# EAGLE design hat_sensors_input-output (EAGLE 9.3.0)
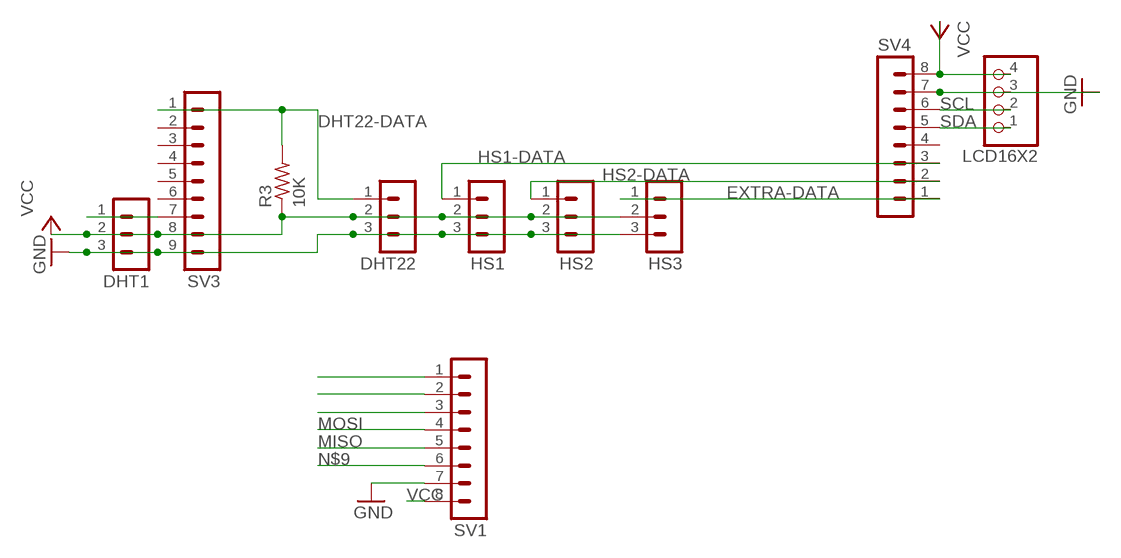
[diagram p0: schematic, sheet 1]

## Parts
DHT1  MA03-1  [MA03-1]
DHT22  MA03-1  [MA03-1]
HS1  MA03-1  [MA03-1]
HS2  MA03-1  [MA03-1]
HS3  MA03-1  [MA03-1]
LCD16X2  PINHD-1X4  [1X04]
R3  10K  RES-US1206  [R1206]
SV1  MA08-1  [MA08-1]
SV3  MA09-1  [MA09-1]
SV4  MA08-1  [MA08-1]

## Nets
DHT22-DATA: DHT22.1 R3.2 SV3.1
EXTRA-DATA: HS3.1 SV4.1
GND: DHT1.3 DHT22.3 HS1.3 HS2.3 HS3.3 LCD16X2.3 SV1.7 SV3.9 SV4.7
HS1-DATA: HS1.1 SV4.3
HS2-DATA: HS2.1 SV4.2
MISO: SV1.5
MOSI: SV1.4
N$2: SV1.1
N$4: DHT1.1 SV3.7
N$9: SV1.6
N$17: SV1.2
N$18: SV1.3
SCL: LCD16X2.2 SV4.6
SDA: LCD16X2.1 SV4.5
VCC: DHT1.2 DHT22.2 HS1.2 HS2.2 HS3.2 LCD16X2.4 R3.1 SV1.8 SV3.8 SV4.8
Unconnected: SV3.2 SV3.3 SV3.4 SV3.5 SV3.6 SV4.4

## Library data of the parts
DHT1 DHT22 HS1-HS3 = con-lstb:MA03-1: PIN HEADER; OC_FARNELL: unknown; OC_NEWARK: unknown
LCD16X2 = pinhead:PINHD-1X4: PIN HEADER
R3 = fab:RES-US: Resistor (US Symbol)
SV1 SV4 = con-lstb:MA08-1: PIN HEADER
SV3 = con-lstb:MA09-1: PIN HEADER; OC_FARNELL: unknown; OC_NEWARK: unknown

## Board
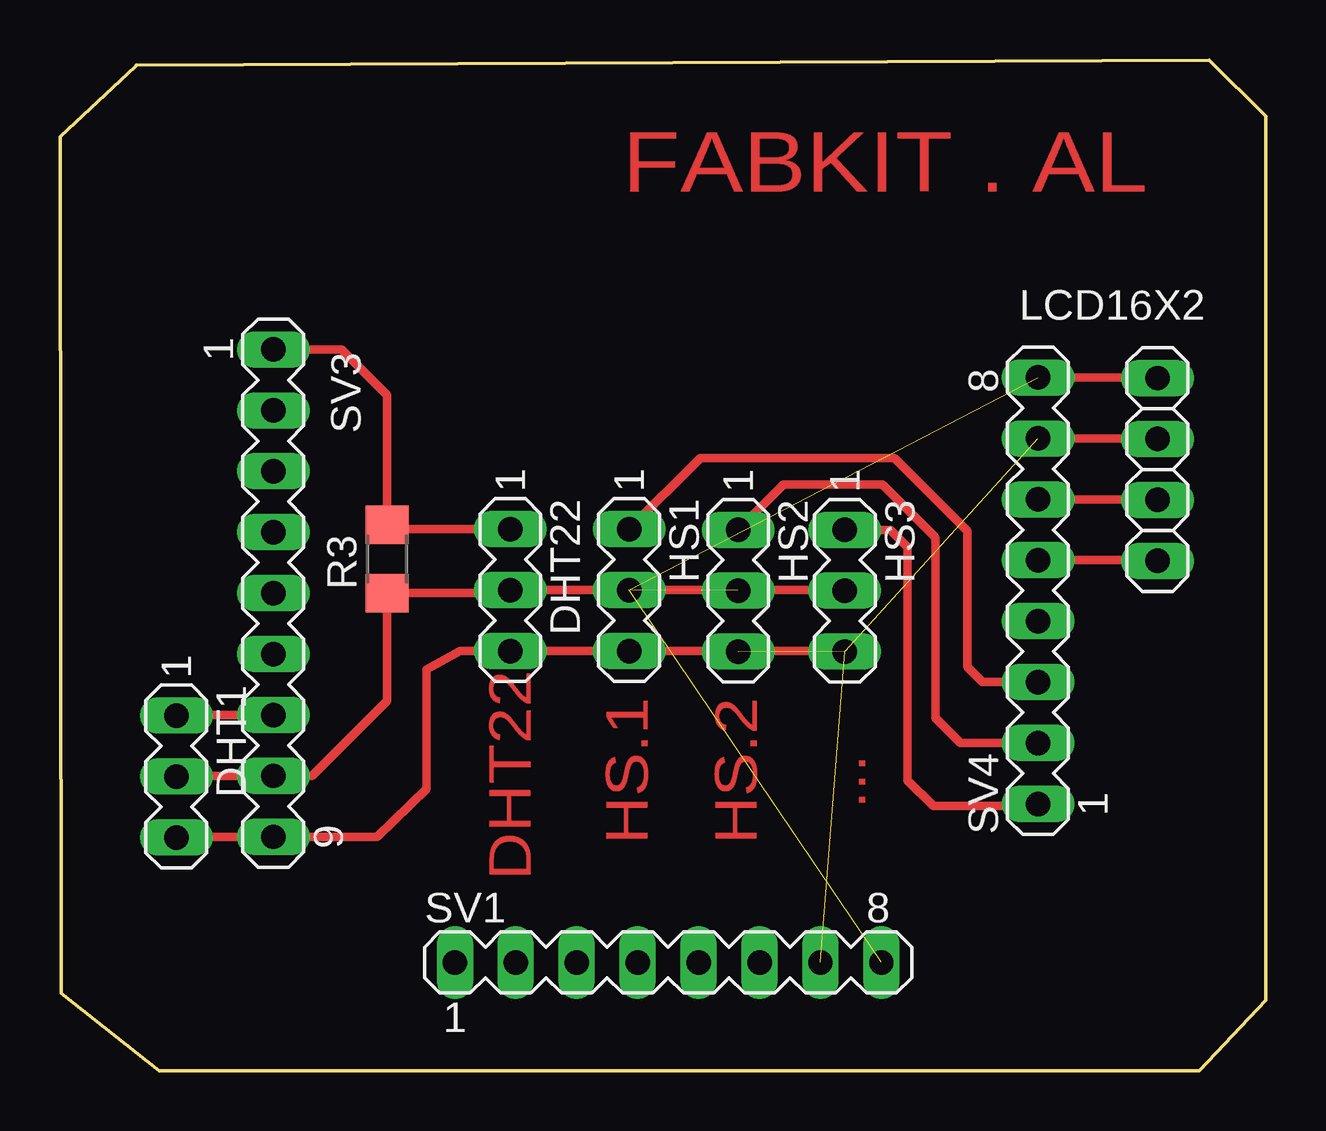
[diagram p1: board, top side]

Size 50.27 x 42.14 mm. Coordinates in mm from the lower left corner, seen from the top.
Outline: 3.15,41.88 0,38.94 0.05,3.23 4.14,0 47.5,0 50.27,2.95 50.27,39.8 47.9,42.14 3.17,41.91
Copper layers (1*16): Top 0.035mm / dielectric 1.5mm / Bottom 0.035mm
Design rules "default *": minimum track width 10mil, minimum drill 24mil, track to track 16mil, track to pad 16mil, pad to pad 16mil, via to via 16mil, smd to smd 16mil, copper to edge 16mil, drill to drill 8mil, minimum pad ring 10mil, minimum via ring 8mil, stop-mask expansion 4mil, vias tented up to drill 0mil, thermal gap 10mil

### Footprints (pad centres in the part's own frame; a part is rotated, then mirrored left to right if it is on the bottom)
MA03-1 = drill 1.016 long: 1 -2.54,0; 2 0,0; 3 2.54,0
1X04 = drill 1.016 long: 1 -3.81,0; 2 -1.27,0; 3 1.27,0; 4 3.81,0
R1206 = smd 1.6 x 1.803: 1 -1.422,0; 2 1.422,0
MA08-1 = drill 1.016 long: 1 -8.89,0; 2 -6.35,0; 3 -3.81,0; 4 -1.27,0; 5 1.27,0; 6 3.81,0; 7 6.35,0; 8 8.89,0
MA09-1 = drill 1.016 long: 1 -10.16,0; 2 -7.62,0; 3 -5.08,0; 4 -2.54,0; 5 0,0; 6 2.54,0; 7 5.08,0; 8 7.62,0; 9 10.16,0

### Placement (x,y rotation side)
DHT1  4.85,12.27 270 top
DHT22  18.77,20.04 270 top
HS1  23.72,20.04 270 top
HS2  28.27,20.02 270 top
HS3  32.72,20.02 270 top
LCD16X2  45.75,25.07 90 top
R3  13.64,21.34 90 top
SV1  25.35,4.52 0 top
SV3  8.89,19.91 270 top
SV4  40.77,20.02 90 top

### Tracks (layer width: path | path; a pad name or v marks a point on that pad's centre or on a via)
DHT22-DATA
  Top 0.356: SV3.1 11.73,30.07 13.64,28.17 R3.2 13.82,22.58 DHT22.1
EXTRA-DATA
  Top 0.356: HS3.1 34.62,22.56 35.33,21.84 35.33,12.12 36.4,11.05 40.69,11.05 SV4.1
GND  (3 unrouted)
  Top 0.356: SV4.7 45.72,26.37 LCD16X2.3 | SV3.9 4.88,9.75 DHT1.3 | SV3.9 8.9,9.74 | HS3.3 32.69,17.5 HS1.3 DHT22.3 16.68,17.5 15.29,16.72 15.29,11.75 13.23,9.75 SV3.9
HS1-DATA
  Top 0.356: HS1.1 26.7,25.55 34.77,25.55 37.82,22.5 37.82,16.84 38.46,16.21 SV4.3
HS2-DATA
  Top 0.356: HS2.1 30.15,24.44 34.29,24.44 36.5,22.23 36.5,14.71 37.54,13.67 SV4.2
N$4
  Top 0.356: SV3.7 4.88,14.83 DHT1.1
SCL
  Top 0.356: SV4.6 45.72,23.83 LCD16X2.2
SDA
  Top 0.356: SV4.5 45.72,21.29 LCD16X2.1
VCC  (3 unrouted)
  Top 0.356: SV4.8 45.72,28.91 LCD16X2.4 | DHT1.2 4.88,12.29 SV3.8 10.52,12.29 13.64,15.42 R3.1 18.64,19.91 DHT22.2 HS1.2 32.69,20.04 HS3.2

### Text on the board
Top: FABKIT . AL | ... | HS.1 | HS.2 | DHT22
